PROGRAM MAIN
VAR
	Axis1	: AXIS_REF;
	
	fbPower	: MC_Power;
	
	fbHome	: FB_NcBasedHoming;
END_VAR


fbPower.Enable			;
fbPower.Enable_Positive	:= TRUE;  
fbPower.Enable_Negative	:= TRUE; 
fbPower( Axis := Axis1 );

fbHome.stParameter.NegativeSwitch := GVL_IO.nDriverDigtalIn.0;
fbHome.stParameter.PositiveSwitch := GVL_IO.nDriverDigtalIn.1;
fbHome.stParameter.RefrenceSignal := GVL_IO.nDriverDigtalIn.2;
fbHome( AxisRef := Axis1 );



//(* 回零模式-寻Z脉冲回零 *)
//fbHome.stParameter.HomeMode 			:= E_HomeMode.ZPULSEHOME;
//(* 回零速度 *)
//fbHome.stParameter.HomeZPulseVelocity	:= 1.0;
//(* 寻Z脉冲方向 *)
//fbHome.stParameter.ZPulseDirection		:= mcNegativeDirection;


//(* 输入负限位信号 *)
//fbHome.stParameter.NegativeSwitch:= GVL_IO.nDriverDigtalIn.0;
//(* 输入正限位信号 *)
//fbHome.stParameter.PositiveSwitch:= GVL_IO.nDriverDigtalIn.1;
//(* 输入原点信号 *)
//fbHome.stParameter.RefrenceSignal:= GVL_IO.nDriverDigtalIn.2;
//(* 回零模式-寻限位开关 *)
//fbHome.stParameter.HomeMode := E_HomeMode.LIMITSWITCH;
//(* 回零速度*)
//fbHome.stParameter.HomeVelocity	:= 1.0;
//(* 回零开始方向-负方向运动 *)
//fbHome.stParameter.StartDirection := MC_Home_Direction.mcNegativeDirection;
//(*原点开关类型-靠近正方向的信号边缘 *)
//fbHome.stParameter.SwitchMode := MC_Switch_Mode.mcRisingEdge;

//(* 附加Z脉冲回零 *)
//fbHome.stParameter.EnableZpulseHome	:= TRUE;
//(* 回零速度 *)
//fbHome.stParameter.HomeZPulseVelocity	:= 1.0;
//(* 寻Z脉冲方向 *)
//fbHome.stParameter.ZPulseDirection		:= mcPositiveDirection;


//(* 回零模式-堵转回零 *)
//fbHome.stParameter.HomeMode := E_HomeMode.BLOCKHOME;
//(* 回零方向 负方向 *)
//fbHome.stParameter.StartDirection	:= MC_Home_Direction.mcNegativeDirection;
//(* 回零速度 *)
//fbHome.stParameter.HomeVelocity		:= 10;
//(* 停转速度限制，低于该值认为停转 *)
//fbHome.stParameter.BlockHomeDetectionVeloLimit	:= 0.5;
//(* 堵转监控时间，超过该时间认为堵转 *)
//fbHome.stParameter.BlockHomeDetectionVeloTime	:= T#100MS;
//(* 移动距离限制，从回零开始起算 *)
//fbHome.stParameter.BlockHomeDistanceLimit		:= 1000;
//(* 跟随误差限制，超过该误差认为堵转 *)
//fbHome.stParameter.BlockHomeLagLimit			:= 10;
//(* 时间限制，开始回零后开始计算，超时报警 *)
//fbHome.stParameter.BlockHomeTimeLimit			:= T#100S;
//(* ！扭矩限值 百分之额定扭矩 *)
//fbHome.stParameter.BlockHomeTorqueLimit			:= 50;


//(* 回零模式 *)
//fbHome.stParameter.HomeMode := E_HomeMode.DIRECTHOME;
//(* 偏置值 *)
//fbHome.stParameter.HomeOffset	:= -150;


//(* 回零模式 *)
//fbHome.stParameter.HomeMode := E_HomeMode.SETPOSITION;
//(* 设定值 *)
//fbHome.stParameter.HomeOffset	:= -150;

END_PROGRAM
